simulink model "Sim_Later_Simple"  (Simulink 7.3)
settings: Solver=ode45  StartTime=0.0  StopTime=20  RelTol=1e-3
InitFcn:
  | init
StartFcn:
  | init
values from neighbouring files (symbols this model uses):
  d2r = pi/180    (= 0.0174532925199)    [init.m]    (also in robust.m)
  r2d = 180/pi    (= 57.2957795131)    [init.m]    (also in robust.m)
undefined symbols (not defined in the file or in its folder): Als, Bls, Cls, Dls, Kmix, Kpr

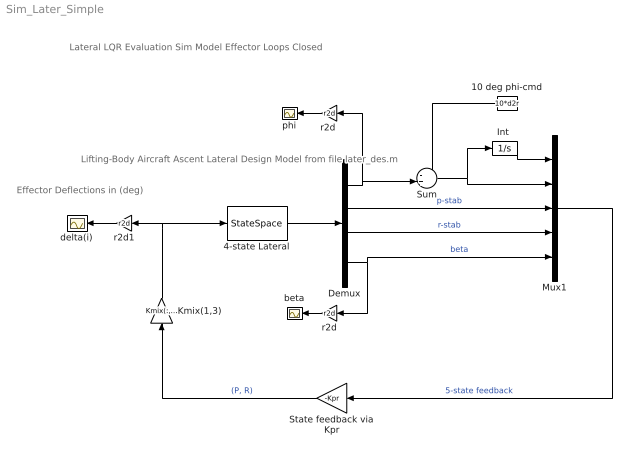
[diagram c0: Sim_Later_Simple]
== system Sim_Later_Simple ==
  note: Lateral LQR Evaluation Sim Model Effector Loops Closed
  note: Effector Deflections in (deg)
  note: Lifting-Body Aircraft Ascent Lateral Design Model from file later_des.m
  10 deg phi-cmd : Constant  Value=10*d2r  OutDataType=sfix(16)  OutScaling=2^0
  4-state Lateral : StateSpace  A=Als  B=Bls  C=Cls  D=Dls
  Demux : Demux
  "Int " : Integrator
  Kmix(1,3) : Gain  Gain=Kmix(:,[1,3])  Multiplication=Matrix(K*u)  ParameterDataType=sfix(16)  ParameterScaling=2^0  OutDataType=sfix(16)  OutScaling=2^0
  Mux1 : Mux  Inputs=5
  State feedback via Kpr : Gain  Gain=-Kpr  Multiplication=Matrix(K*u)  ParameterDataType=sfix(16)  ParameterScaling=2^0  OutDataType=sfix(16)  OutScaling=2^0
  Sum : Sum  Inputs=-+|  OutDataType=sfix(16)  OutScaling=2^0
  beta : Scope
  delta(i) : Scope
  phi : Scope
  r2d : Gain  Gain=r2d  ParameterDataType=sfix(16)  ParameterScaling=2^0  OutDataType=sfix(16)  OutScaling=2^0
  "r2d " : Gain  Gain=r2d  ParameterDataType=sfix(16)  ParameterScaling=2^0  OutDataType=sfix(16)  OutScaling=2^0
  r2d1 : Gain  Gain=r2d  ParameterDataType=sfix(16)  ParameterScaling=2^0  OutDataType=sfix(16)  OutScaling=2^0
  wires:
  4-state Lateral/1 -> Demux/1
  Demux/2 -> Mux1/3  "p-stab"
  Demux/3 -> Mux1/4  "r-stab"
  Demux/4 -> Mux1/5, r2d/1  "beta"
  Mux1/1 -> State feedback via Kpr/1  "5-state feedback"
  State feedback via Kpr/1 -> Kmix(1,3)/1  "(P, R)"
  Kmix(1,3)/1 -> r2d1/1, 4-state Lateral/1
  r2d1/1 -> delta(i)/1
  Sum/1 -> Mux1/2, "Int "/1
  Demux/1 -> Sum/2, "r2d "/1
  "Int "/1 -> Mux1/1
  10 deg phi-cmd/1 -> Sum/1
  "r2d "/1 -> phi/1
  r2d/1 -> beta/1
